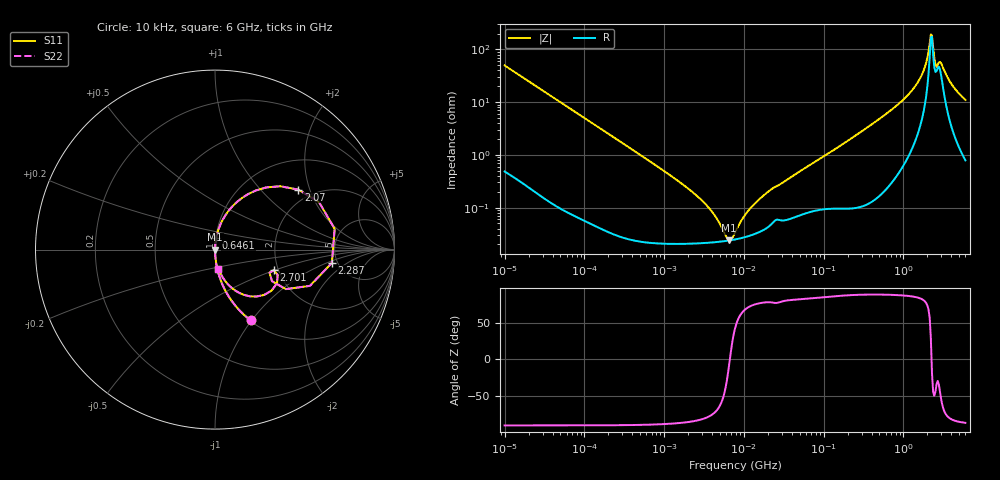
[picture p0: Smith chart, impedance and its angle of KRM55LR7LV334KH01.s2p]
!Murata Part Number: KRM55LR7LV334KH01
!These Parameters are Measured in Series Mode Connection
!Data Generated on Jan 08, 2026
!  o--ll--o
!Port1  Port2
!  o------o
!Operation Temp=25[degC], DC Bias Voltage=0[V]
!Freq. Start=10[kHz] Stop=6[GHz] 401[Steps]
# Hz S RI R 50
!Freq.(Hz) S11(Real) S11(Imag) S21(Real) S21(Imag) S12(Real) S12(Imag) S22(Real) S22(Imag)
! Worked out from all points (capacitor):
!   401 points, 10 kHz to 6 GHz, reference 50 ohm
!   read as one part in series: C = 321 nF near 10.69 kHz
!   lowest |Z| = 24 mohm at 6.559 MHz (marker M1)
!   series resonance near 6.671 MHz, so ESL is about 1.8 nH
!   S11 on the Smith chart (normalised r, x): 10 kHz: 1.01, -0.99; 646.1 MHz: 1.00, +0.13; 2.07 GHz: 1.69, +1.68; 2.287 GHz: 4.49, -1.16; 2.701 GHz: 1.89, -0.49; 6 GHz: 1.02, -0.22
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10000  0.1995 -0.3948  0.8005 0.3948  0.8005 0.3948  0.1995 -0.3948
22969  0.0468 -0.2064  0.9532 0.2064  0.9532 0.2064  0.0468 -0.2064
92862  0.0035 -0.0538  0.9965 0.0538  0.9965 0.0538  0.0035 -0.0538
862344  0.000242 -0.00575  0.9998 0.00575  0.9998 0.00575  0.000242 -0.00575
3155371  0.000215 -0.00123  0.9998 0.00123  0.9998 0.00123  0.000215 -0.00123
4256561  0.000221 -0.000697  0.9998 0.000697  0.9998 0.000697  0.000221 -0.000697
6559168  0.000238 -2.51e-05  0.9998 2.51e-05  0.9998 2.51e-05  0.000238 -2.51e-05
7745967  0.000249 0.000224  0.9998 -0.000224  0.9998 -0.000224  0.000249 0.000224
1.044922e7  0.000277 0.000687  0.9997 -0.000687  0.9997 -0.000687  0.000277 0.000687
1.610178e7  0.000353 0.00146  0.9996 -0.00146  0.9996 -0.00146  0.000353 0.00146
7.193098e7  0.00089 0.00676  0.9991 -0.00676  0.9991 -0.00676  0.00089 0.00676
6.461166e8  0.00652 0.0635  0.9935 -0.0635  0.9935 -0.0635  0.00652 0.0635
6.67969e8  0.00699 0.066  0.993 -0.066  0.993 -0.066  0.00699 0.066
1.58612e9  0.0895 0.2326  0.9105 -0.2326  0.9105 -0.2326  0.0895 0.2326
1.811831e9  0.1826 0.3082  0.8174 -0.3082  0.8174 -0.3082  0.1826 0.3082
2.069661e9  0.4649 0.334  0.5351 -0.334  0.5351 -0.334  0.4649 0.334
2.286837e9  0.6512 -0.0739  0.3488 0.0739  0.3488 0.0739  0.6512 -0.0739
2.44414e9  0.3944 -0.2203  0.6056 0.2203  0.6056 0.2203  0.3944 -0.2203
2.700612e9  0.327 -0.1149  0.673 0.1149  0.673 0.1149  0.327 -0.1149
3.297118e9  0.1925 -0.2599  0.8075 0.2599  0.8075 0.2599  0.1925 -0.2599
4.025378e9  0.0731 -0.1943  0.9269 0.1943  0.9269 0.1943  0.0731 -0.1943
6e9  0.0194 -0.1065  0.9806 0.1065  0.9806 0.1065  0.0194 -0.1065
